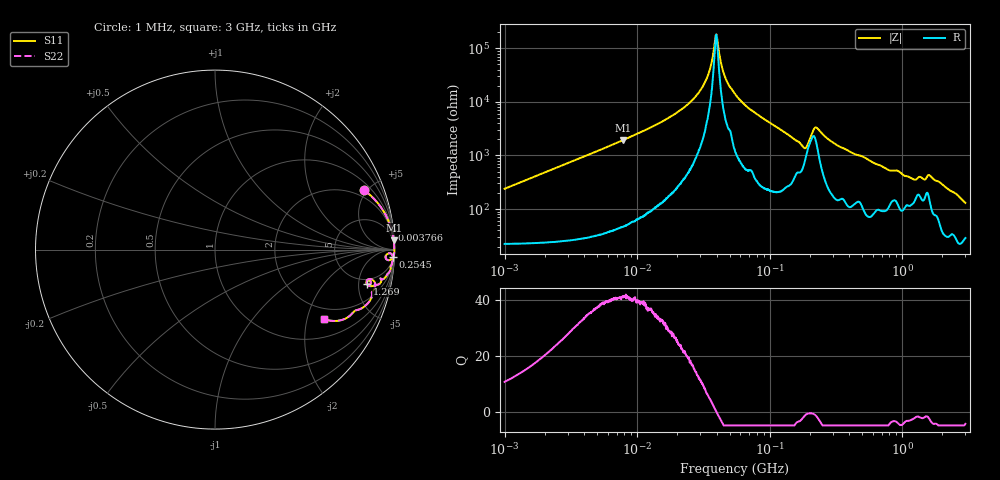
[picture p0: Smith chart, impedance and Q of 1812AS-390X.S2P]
!s-Parameter Generated by FASTRON Sdn. Bhd.
!FASTRON P/N : 1812AS-390X
!Keysight Technologies,E4991B,MY54100416,A.01.15
!Date created: Mon Oct 16 10:08:21 2023
!Version  : Rev00 Mon Oct 16 10:08:21 2023
!Data & Calibration Information:
!Freq	S11	S21	S12	S22
!PortZ  Port1:50+j0  Port2:50+j0
!When reading, reference impedance value at option line is always used.
! Remarks : This data is being provided solely for informational purposes.
# Hz S dB R 50
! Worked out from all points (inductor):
!   1601 points, 1 MHz to 3 GHz, reference 50 ohm
!   read as one part in series: L = 37.8 uH near 1.041 MHz
!   highest Q = 41.2 at 7.82 MHz (marker M1), where L = 39.2 uH
!   self-resonance near 39.37 MHz
!   S11 on the Smith chart (normalised r, x): 1 MHz: 1.45, +4.76; 3.766 MHz: 2, +18; 254.5 MHz: 9, -48; 1.269 GHz: 4.17, -6.34; 3 GHz: 1.58, -2.54
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1000000  -0.98 21.8  -8.55 -62.8  -8.55 -62.8  -0.98 21.8
3766155  -0.08 6.3  -19.19 -81.9  -19.19 -81.9  -0.08 6.3
3804036  -0.08 6.2  -19.28 -82.0  -19.28 -82.0  -0.08 6.2
7819618  -0.02 3.0  -25.72 -85.7  -25.72 -85.7  -0.02 3.0
1.447069e7  -0.01 1.5  -31.92 -86.8  -31.92 -86.8  -0.01 1.5
2.247661e7  -0.01 0.7  -37.84 -86.6  -37.84 -86.6  -0.01 0.7
2.959763e7  -0.00 0.4  -43.90 -84.7  -43.90 -84.7  -0.00 0.4
3.473756e7  -0.00 0.2  -50.82 -78.9  -50.82 -78.9  -0.00 0.2
3.936673e7  -0.00 0.0  -65.12 -10.9  -65.12 -10.9  -0.00 0.0
4.05666e7  -0.00 -0.0  -62.10 46.2  -62.10 46.2  -0.00 -0.0
4.574308e7  -0.01 -0.2  -49.71 79.3  -49.71 79.3  -0.01 -0.2
5.477226e7  -0.01 -0.4  -42.95 84.7  -42.95 84.7  -0.01 -0.4
7.034296e7  -0.01 -0.8  -37.40 85.2  -37.40 85.2  -0.01 -0.8
1.802115e8  -0.29 -3.5  -23.29 59.7  -23.29 59.7  -0.29 -3.5
2.083556e8  -0.28 -1.2  -28.32 32.7  -28.32 32.7  -0.28 -1.2
2.245966e8  -0.14 -1.4  -30.56 56.8  -30.56 56.8  -0.14 -1.4
2.545267e8  -0.07 -2.3  -27.72 77.6  -27.72 77.6  -0.07 -2.3
7.925923e8  -0.46 -10.0  -14.99 68.2  -14.99 68.2  -0.46 -10.0
1.268618e9  -1.24 -12.6  -12.23 50.8  -12.23 50.8  -1.24 -12.6
1.604986e9  -0.85 -11.4  -13.49 58.2  -13.49 58.2  -0.85 -11.4
2.081985e9  -0.91 -19.6  -9.44 63.4  -9.44 63.4  -0.91 -19.6
3e9  -2.85 -32.6  -5.15 44.6  -5.15 44.6  -2.85 -32.6
